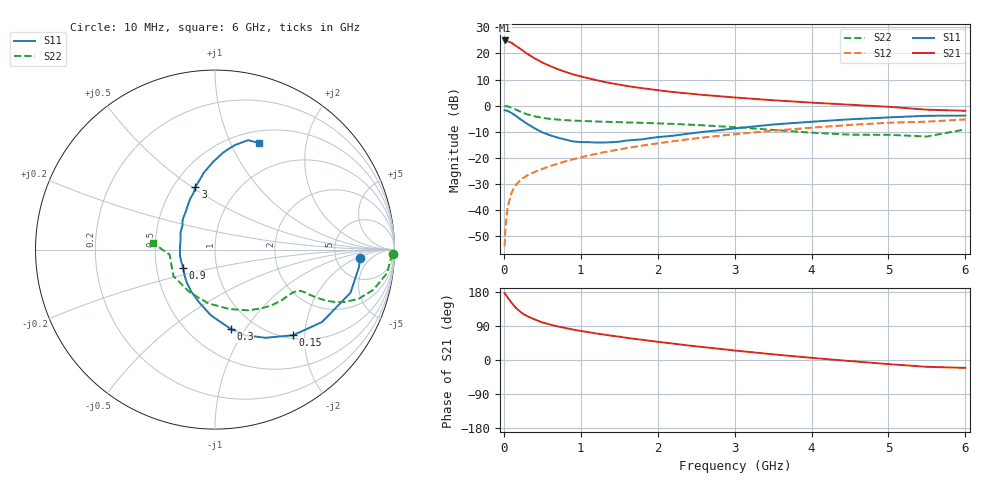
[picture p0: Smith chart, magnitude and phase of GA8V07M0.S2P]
! Infineon Technologies  Discrete & RF Semiconductors
! BF775
! Si NPN RF Bipolar Junction Transistor in SOT23
! VCE = 8 V  IC = 7 mA
! Common Emitter S-Parameters:  May  1996
# GHz  S  MA  R  50
!  f  S11  S21  S12  S22
! GHz  MAG  ANG  MAG  ANG  MAG  ANG  MAG  ANG
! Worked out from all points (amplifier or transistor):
!   36 points, 10 MHz to 6 GHz, reference 50 ohm
!   highest |S21| = 25.0 dB at 10 MHz (marker M1)
!   |S21| within 3 dB of that: start of sweep to 204.9 MHz
!   unconditionally stable (mu >= 1): 739.6 MHz to 2.927 GHz
!   at 250 MHz: K = 0.56, MSG = 24.4 dB, |S12| = -27.8 dB
!   at 1.4 GHz: K = 1.10, MAG = 11.0 dB, |S12| = -17.4 dB
!   at 6 GHz: K = 0.90, MSG = 1.7 dB, |S12| = -5.3 dB
!   S11 on the Smith chart (normalised r, x): 10 MHz: 8.78, -2.52; 150 MHz: 1.07, -1.75; 300 MHz: 0.77, -0.86; 900 MHz: 0.69, -0.15; 3 GHz: 0.64, +0.51; 6 GHz: 0.64, +1.28
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0.01  0.8098 -3.5  17.79 176.6  0.002 92.8  0.9913 -1.5
0.02  0.8081 -6.8  17.43 173.4  0.0044 84.7  0.981 -3.1
0.05  0.7925 -17.6  17.16 164.8  0.0113 79.8  0.9672 -7.8
0.1  0.7206 -34.0  16.03 151.2  0.0211 74.4  0.9096 -14.3
0.15  0.6458 -47.6  14.21 139.1  0.0291 68.1  0.8448 -19.0
0.2  0.5669 -60.1  12.75 129.7  0.0353 64.5  0.782 -21.9
0.25  0.5062 -70.6  11.27 122.0  0.0406 61.9  0.7251 -23.7
0.3  0.45 -78.9  9.954 116.1  0.0453 61.8  0.6817 -24.7
0.4  0.3664 -93.7  8.072 107.1  0.0533 60.5  0.6227 -25.3
0.5  0.3058 -107.1  6.701 99.3  0.0607 60.8  0.5814 -25.5
0.6  0.2697 -119.1  5.745 93.6  0.0691 61.5  0.5558 -25.4
0.7  0.2424 -130.3  5.011 88.7  0.0767 62.1  0.5387 -25.6
0.9  0.2049 -149.6  3.979 80.3  0.0931 62.5  0.5157 -26.5
1.1  0.198 -170.1  3.338 73.4  0.11 63.1  0.5009 -28.2
1.3  0.1955 174.3  2.86 67.1  0.127 62.5  0.4891 -30.2
1.6  0.2136 154.4  2.377 58.4  0.1528 61.2  0.4753 -34.0
2.2  0.2639 128.7  1.818 43.2  0.207 57.4  0.445 -43.7
3  0.3644 107.4  1.431 25.1  0.2823 50.2  0.3859 -61.2
3.5  0.4328 98.3  1.266 14.9  0.3291 44.7  0.3409 -76.3
4.5  0.5452 84.9  1.038 -2.8  0.4254 32.5  0.2766 -121.1
5.5  0.6373 73.1  0.834 -18.0  0.4912 17.4  0.2548 -173.8
6  0.642 67.7  0.794 -20.8  0.5418 13.2  0.3495 173.7
